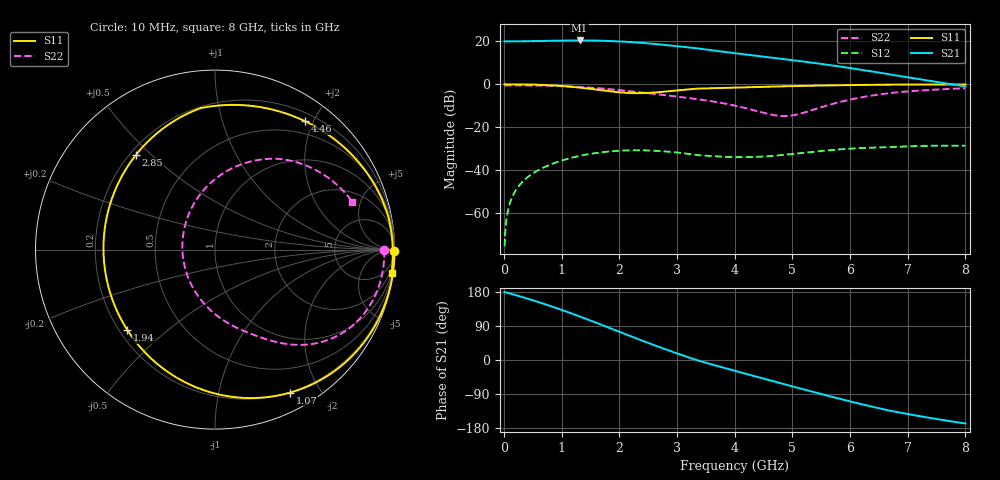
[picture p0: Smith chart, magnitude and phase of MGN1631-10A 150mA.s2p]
! Port[1] = GATE
! Port[2] = DRAIN
! [Type]  S-parameter s2p file touchstone ver. 1.0
! [Object]  MGN1631-10A
! [Bias]  150 mA
! [Version]  1.0
! [Date]  Thu May 19 10:54:03 2026
! [Source]  This file was created in JSC "ICC Milandr".
! [Disclaimer] Property of JSC "ICC Milandr". Unauthorized reproduction and/or distribution is strictly prohibited.
!  The file and the data are provided "AS IS" and with all faults and disclaim all warranties, express and implied, including
!  without limitation any implied warranties of merchantability, fitness for a particular purpose.
!  JSC "ICC Milandr" assumes no liability for:
!  1) the accuracy of the data provided;
!  2) the proper functioning of this data;
!  3) infringement of patents, copyrights or intellectual property rights resulting from the use of this data.
!  JSC "ICC Milandr" reserves the right to make changes to the products and the data without prior notice.
!  Please, be aware that your receipt and use of the file provided shall serve as acceptance of these terms and conditions.
!  If you do not accept these terms, you should return or destroy this file and any other accompanying information immediately.
# Hz S MA R 12.5
! freq  S11mag  S11ang  S21mag  S21ang  S12mag  S12ang  S22mag  S22ang
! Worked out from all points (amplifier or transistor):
!   800 points, 10 MHz to 8 GHz, reference 12.5 ohm
!   highest |S21| = 20.5 dB at 1.31 GHz (marker M1)
!   |S21| within 3 dB of that: start of sweep to 3.119 GHz
!   unconditionally stable (mu >= 1): 3.508 GHz to 4.714 GHz
!   at 1.34 GHz: K = 0.39, MSG = 26.9 dB, |S12| = -33.2 dB
!   at 4.01 GHz: K = 1.13, MAG = 22.1 dB, |S12| = -34.0 dB
!   at 8 GHz: K = 0.27, MSG = 13.8 dB, |S12| = -28.6 dB
!   S11 on the Smith chart (normalised r, x): 10 MHz: open; 1.07 GHz: 0.20, -1.64; 1.94 GHz: 0.23, -0.37; 2.85 GHz: 0.22, +0.45; 4.46 GHz: 0.31, +1.88; 8 GHz: 1, -15
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1e7  1 -0.5  10.06 179.4  0.0001669 85.1  0.9437 -0.2
1.7e8  0.9996 -8.9  10.06 172.6  0.002814 83.7  0.9438 -3.7
5.8e8  0.9789 -31.4  10.25 153.7  0.009675 68.5  0.935 -12.9
8.3e8  0.947 -46.4  10.4 141.2  0.01386 58.2  0.9208 -18.7
1.07e9  0.9003 -62.2  10.52 128.4  0.01776 47.7  0.899 -24.4
1.31e9  0.8388 -79.8  10.57 115.1  0.02136 36.7  0.8681 -30.2
1.35e9  0.8274 -82.9  10.56 112.8  0.02191 34.8  0.8621 -31.1
1.65e9  0.7383 -108.6  10.44 95.3  0.02552 20.4  0.8091 -38.3
1.94e9  0.6629 -137.4  10.12 78.0  0.02784 6.3  0.7478 -44.8
2.32e9  0.6214 -178.7  9.428 55.5  0.02886 -11.7  0.6613 -52.7
2.68e9  0.6552 144.7  8.582 34.8  0.02783 -27.7  0.582 -59.6
2.85e9  0.6874 129.8  8.154 25.4  0.02679 -34.6  0.5469 -63.0
3.1e9  0.7413 111.0  7.526 12.1  0.02476 -44.1  0.498 -68.3
3.38e9  0.7949 93.9  6.83 -2.0  0.02218 -52.7  0.4454 -75.5
3.68e9  0.8169 80.5  6.038 -15.1  0.02083 -55.6  0.3861 -85.0
4.01e9  0.8416 68.4  5.313 -28.9  0.02003 -55.2  0.3165 -99.1
4.46e9  0.8738 54.9  4.495 -47.5  0.02053 -50.8  0.2232 -129.9
4.88e9  0.9014 44.5  3.844 -64.7  0.02274 -46.2  0.1817 179.8
5.34e9  0.9285 34.5  3.207 -83.4  0.02642 -43.9  0.2498 124.9
5.98e9  0.9594 22.2  2.422 -108.5  0.03138 -46.0  0.4338 82.9
6.67e9  0.9829 10.6  1.724 -133.1  0.03377 -51.9  0.6201 54.6
8e9  0.9926 -7.5  0.8957 -167.6  0.03696 -77.9  0.8095 19.3
